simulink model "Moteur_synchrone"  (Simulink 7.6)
settings: Solver=ode23tb  StartTime=0.0  StopTime=2  RelTol=1e-4
InitFcn:
  | clc
  | close all
  | clear all
StopFcn:
  | load vitesse.mat
  | plotyy(x(1,:), x(2,:), x(1,:), x(3,:))
  | grid
  | title('Position et Vitesse de rotation du rotor (rad/s)')
  | xlabel('temps')
  | 
  | delete *.mat, clear all
libraries: powerlib x5, powerlib_extras x1

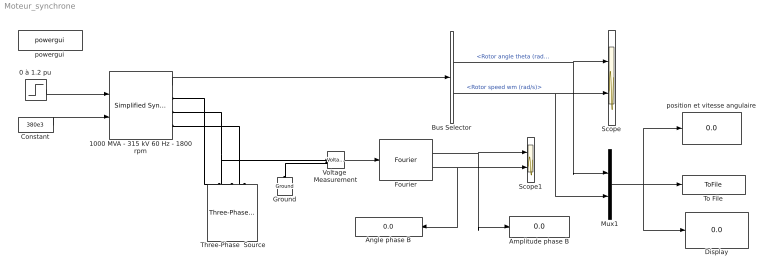
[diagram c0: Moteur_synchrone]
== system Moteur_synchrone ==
  " Three-Phase  Source" : powerlib/Electrical Sources/Three-Phase Source  DialogController=POWERSYS.PowerSysDialog  SystemSampleTime=-1  Voltage=380e3  PhaseAngle=0  Frequency=60  InternalConnection=Yg  SpecifyImpedance=off  Resistance=0  Inductance=0  ShortCircuitLevel=100e6  BaseVoltage=25e3  XRratio=7
  0 à 1.2 pu : Step  After=1.2*1e9  SampleTime=0
  1000 MVA - 315 kV 60 Hz - 1800 rpm : powerlib/Machines/Simplified Synchronous Machine SI Units  DialogController=POWERSYS.PowerSysDialog  SystemSampleTime=-1  ConnectionType=3-wire Y  MechanicalLoad=Mechanical power Pm  NominalParameters=[1000e6, 380e3, 60 ]  Mechanical="[10e6,  80,  20]"  InternalRL=[0.5 , 0.03]  InitialConditions=[0 5 1e3 1e3 1e3 0 -120 120]  Units=1  LoadFlowParameters=[1 500000000 0 0 0]  TsPowergui=0  TsBlock=-1
  Amplitude phase B : Display
  Angle phase B : Display
  Bus Selector : BusSelector  OutputSignals=Rotor angle theta (rad),Rotor speed wm (rad/s)
  Constant : Constant  Value=380e3
  Display : Display
  Fourier : powerlib_extras/Measurements/Fourier  DialogController=POWERSYS.PowerSysDialog  SystemSampleTime=-1  f1=60  n=1
  Ground : powerlib/Elements/Ground  DialogController=POWERSYS.PowerSysDialog  PhysicalDomain=powersysdomain  SubClassName=unknown  LeftPortType=p1  RightPortType=p1  LConnTagsString=a
  Mux1 : Mux  Inputs=2
  Scope : Scope  NumInputPorts=2
  Scope1 : Scope  NumInputPorts=2
  To File : ToFile  Filename=vitesse  MatrixName=x
  Voltage  Measurement : powerlib/Measurements/Voltage Measurement  DialogController=POWERSYS.PowerSysDialog  SystemSampleTime=-1  PhasorSimulation=off  OutputType=Complex  PSBequivalent=0
  position et vitesse angulaire : Display
  powergui : powerlib/powergui  Priority=2  SystemSampleTime=-1  SimulationMode=Continuous  SampleTime=1e-5  frequency=60  SPID=off  DisableSnubberDevices=off  DisableRonSwitches=off  DisableVfSwitches=off  SwTol=0  Interpol=off  frequencyindice=60  echomessages=off  HookPort=off  DisplayEquations=off  FunctionMessages=off  EnableUseOfTLC=off  x0status=blocks  RestoreLinks=warning  ResistiveCurrentMeasurement=off  Frange=logspace(0,3,50)  Ylog=off  Xlog=off  ShowGrid=off  save=off  variable=ZData  ZoomFFT=on  StartTime=0.0  cycles=2  DisplayStyle=off  fundamental=60  FreqAxis=off  MaxFrequency=1000  frequencyindicesteady=1  RmsSteady=1  display=off  Ts=0  methode=off
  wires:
  1000 MVA - 315 kV 60 Hz - 1800 rpm/1 -> Bus Selector/1
  0 à 1.2 pu/1 -> 1000 MVA - 315 kV 60 Hz - 1800 rpm/1
  Constant/1 -> 1000 MVA - 315 kV 60 Hz - 1800 rpm/2
  Bus Selector/1 -> Scope/1, Mux1/1  "<Rotor angle theta (rad)>"
  Bus Selector/2 -> Scope/2, Mux1/2  "<Rotor speed wm (rad/s)>"
  Mux1/1 -> To File/1, position et vitesse angulaire/1, Display/1
  Voltage  Measurement/1 -> Fourier/1
  Fourier/1 -> Scope1/1, Amplitude phase B/1
  Fourier/2 -> Scope1/2, Angle phase B/1
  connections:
  1000 MVA - 315 kV 60 Hz - 1800 rpm/RConn1 -- " Three-Phase  Source"/RConn1
  1000 MVA - 315 kV 60 Hz - 1800 rpm/RConn2 -- " Three-Phase  Source"/RConn2 -- Voltage  Measurement/LConn1
  1000 MVA - 315 kV 60 Hz - 1800 rpm/RConn3 -- " Three-Phase  Source"/RConn3
  Ground/LConn1 -- Voltage  Measurement/LConn2
